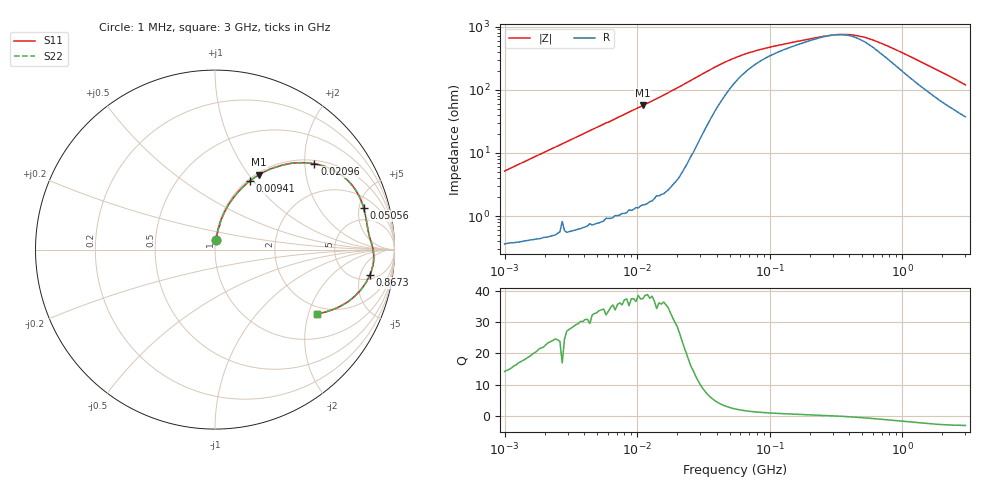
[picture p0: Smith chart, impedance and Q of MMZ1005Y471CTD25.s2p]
! S-Parameter Data Generated by TDK Corporation
! Copyright(C) 2025 TDK Corporation.
! All Rights Reserved.
! TDK P/N: MMZ1005Y471CTD25 (Chip Bead)
! Property: |Z|=470ohm at 100MHz
! Size(LxWxT): 1x0.5x0.5mm
! Model Type: s2p (Touchstone File Format Version 1.0)
! Frequency: DC=Yes Start=1MHz Stop=3000MHz 202points Log-sweep
! Model Generated on Feb. 6, 2025
! Terms and conditions regarding TDK Simulation Models:
! 1)This simulation model is being provided solely for informational
!  purposes. Please refer to the specifications of the products in
!  terms of detailed characteristics of such products.
! 2)In no event shall TDK Corporation of any of its subsidiaries be
!  liable for any loss or damage arising, directly or indirectly,
!  from any information contained in this simulation model, including,
!  but not limited to loss or damages arising from any inaccuracies,
!  omissions or errors in connection with such information.
! 3)Any and all copyrights on this simulation model are owned by
!  TDK Corporation.  Duplication or redistribution of this simulation
!  model without prior written permission from TDK Corporation
!  is prohibited.
! 4)This simulation model is subject to any modification or change
!  without any prior notice.
! 5)Neither TDK Corporation nor any of its subsidiaries shall make any
!  warranty, express or implied, including but not limited to the
!  correctness, implied warranties of merchantability and fitness for
!  a particular purpose with respect to this simulation models.
! 6)The use of this simulation model shall be deemed to have consented
!  to the terms and conditions hereof.
! Port Assignments:
!  1 ---@@@--- 2
! Applicable Conditions:
!  Temperature = 25 degC
!  DC Bias Current = 0 A
!  Small Signal Operation
# Hz S MA R 50
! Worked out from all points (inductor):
!   201 points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, 1 MHz to 3 GHz, reference 50 ohm
!   read as one part in series: L = 818 nH near 1.041 MHz
!   highest Q = 38.5 at 11.04 MHz (marker M1), where L = 810 nH
!   self-resonance near 312 MHz
!   S11 on the Smith chart (normalised r, x): 1 MHz: 1.01, +0.10; 9.41 MHz: 1.03, +0.96; 20.96 MHz: 1.08, +2.23; 50.56 MHz: 3.13, +5.57; 867.3 MHz: 6.05, -7.29; 3 GHz: 1.74, -2.26
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1000000  0.05126 83.0  0.9951 -2.9  0.9951 -2.9  0.05126 83.0
2055611  0.1043 81.5  0.99 -6.0  0.99 -6.0  0.1043 81.5
3900413  0.1939 76.9  0.9746 -11.2  0.9746 -11.2  0.1939 76.9
6305767  0.3014 70.8  0.9448 -17.5  0.9448 -17.5  0.3014 70.8
9410094  0.427 63.2  0.893 -25.3  0.893 -25.3  0.427 63.2
1.104425e7  0.4847 59.5  0.8619 -29.0  0.8619 -29.0  0.4847 59.5
1.461624e7  0.5935 52.0  0.7886 -36.4  0.7886 -36.4  0.5935 52.0
2.095589e7  0.7317 40.8  0.6544 -47.0  0.6544 -47.0  0.7317 40.8
3.254976e7  0.839 26.4  0.4481 -56.3  0.4481 -56.3  0.839 26.4
5.055795e7  0.8602 15.6  0.2883 -53.5  0.2883 -53.5  0.8602 15.6
5.477226e7  0.8598 14.2  0.2688 -51.7  0.2688 -51.7  0.8598 14.2
9.216659e7  0.8587 7.9  0.1902 -38.2  0.1902 -38.2  0.8587 7.9
2.136344e8  0.8722 2.4  0.1336 -15.7  0.1336 -15.7  0.8722 2.4
3.062963e8  0.8806 0.1  0.1194 -0.9  0.1194 -0.9  0.8806 0.1
4.219165e8  0.8853 -2.2  0.1203 16.4  0.1203 16.4  0.8853 -2.2
5.364635e8  0.8859 -4.2  0.1337 29.3  0.1337 29.3  0.8859 -4.2
8.005644e8  0.8778 -8.4  0.1834 44.2  0.1834 44.2  0.8778 -8.4
8.672962e8  0.8744 -9.3  0.1972 46.0  0.1972 46.0  0.8744 -9.3
1.243477e9  0.8497 -14.3  0.2744 49.9  0.2744 49.9  0.8497 -14.3
1.712864e9  0.8093 -19.8  0.3636 49.0  0.3636 49.0  0.8093 -19.8
2.266846e9  0.7521 -25.6  0.4576 45.3  0.4576 45.3  0.7521 -25.6
3e9  0.6697 -32.3  0.5626 39.5  0.5626 39.5  0.6697 -32.3
